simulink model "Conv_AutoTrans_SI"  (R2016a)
settings: Solver=FixedStepDiscrete  StartTime=0.0  StopTime=150  FixedStep=0.05  RelTol=1e-3
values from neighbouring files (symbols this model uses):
  VM = 1400    [initVehicle.m]
  WR = 0.25    [initVehicle.m]    (also in initWheel.m)
undefined symbols (not defined in the file or in its folder): Torque
libraries: libAutoTrans x3, libEngine x2, libWheel x1

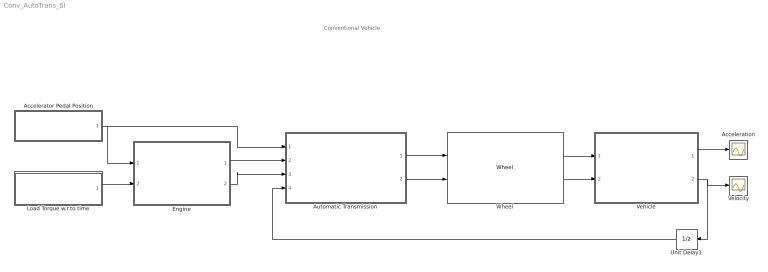
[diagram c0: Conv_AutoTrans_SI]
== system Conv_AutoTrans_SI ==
  note: Conventional Vehicle
  Acceleration : Scope
  Accelerator Pedal Position : Subsystem
  Automatic Transmission : Subsystem
  Engine : Subsystem
  Load Torque w.r.to time : Subsystem
  Unit Delay1 : UnitDelay  SampleTime=-1
  Vehicle : Subsystem
  Velocity : Scope
  Wheel : libWheel/Wheel
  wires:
  Wheel/1 -> Vehicle/1(wheel_speed)
  Wheel/2 -> Vehicle/2(propulsive_force)
  Load Torque w.r.to time/1(load_vs_time) -> Engine/2(load_vs_time)
  Vehicle/2(vehicle_velocity) -> Velocity/1, Unit Delay1/1
  Accelerator Pedal Position/1(pedal_position) -> Automatic Transmission/1(throttle_pos), Engine/1(throttle_position)
  Automatic Transmission/1(trans_speed) -> Wheel/1
  Automatic Transmission/2(trans_torque) -> Wheel/2
  Engine/1(eng_speed) -> Automatic Transmission/2(eng_speed)
  Engine/2(eng_torque) -> Automatic Transmission/3(eng_torque)
  Vehicle/1(vehicle_acceleration) -> Acceleration/1
  Unit Delay1/1 -> Automatic Transmission/4(vehicle_speed)

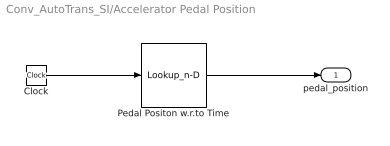
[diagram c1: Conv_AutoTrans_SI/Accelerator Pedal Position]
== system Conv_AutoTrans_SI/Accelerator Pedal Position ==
  Clock : Clock
  Pedal Positon w.r.to Time : Lookup_n-D  NumberOfTableDimensions=1  BreakpointsForDimension1=[0,20,25,35,40,60,65,75,80,100,105,115,120,140,145,155,160,180,185,195,200]  Table=[10,10,80,80,10,10,80,80,10,10,80,80,10,10,80,80,10,10,80,80,10]  RndMeth=Simplest
  pedal_position : Outport
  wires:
  Pedal Positon w.r.to Time/1 -> pedal_position/1
  Clock/1 -> Pedal Positon w.r.to Time/1

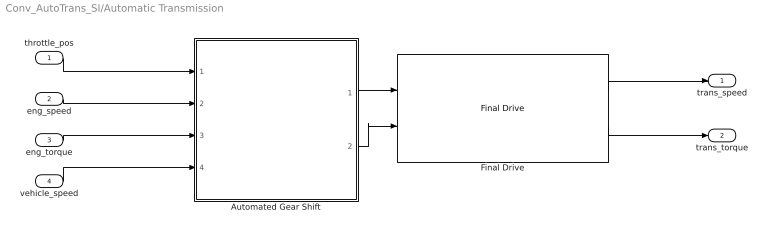
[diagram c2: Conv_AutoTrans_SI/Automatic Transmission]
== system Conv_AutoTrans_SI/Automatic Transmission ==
  throttle_pos : Inport
  eng_speed : Inport  Port=2
  eng_torque : Inport  Port=3
  vehicle_speed : Inport  Port=4
  Automated Gear Shift : Subsystem
  Final Drive : libAutoTrans/Final Drive
  trans_speed : Outport
  trans_torque : Outport  Port=2
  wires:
  Final Drive/1 -> trans_speed/1
  Final Drive/2 -> trans_torque/1
  Automated Gear Shift/1(speed_output) -> Final Drive/1
  Automated Gear Shift/2(torque_output) -> Final Drive/2
  throttle_pos/1 -> Automated Gear Shift/1(throttle_pos)
  eng_speed/1 -> Automated Gear Shift/2(eng_speed)
  eng_torque/1 -> Automated Gear Shift/3(eng_torque)
  vehicle_speed/1 -> Automated Gear Shift/4(vehicle_speed)

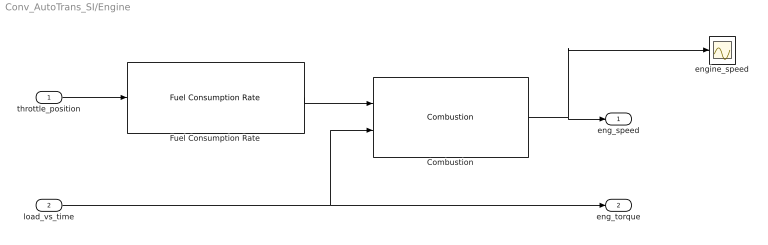
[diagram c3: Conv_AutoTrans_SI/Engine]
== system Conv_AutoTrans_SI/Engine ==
  throttle_position : Inport
  load_vs_time : Inport  Port=2
  Combustion : libEngine/Combustion
  Fuel Consumption Rate : libEngine/Fuel Consumption Rate
  engine_speed : Scope
  eng_speed : Outport
  eng_torque : Outport  Port=2
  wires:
  throttle_position/1 -> Fuel Consumption Rate/1
  Fuel Consumption Rate/1 -> Combustion/1
  load_vs_time/1 -> Combustion/2, eng_torque/1
  Combustion/1 -> engine_speed/1, eng_speed/1

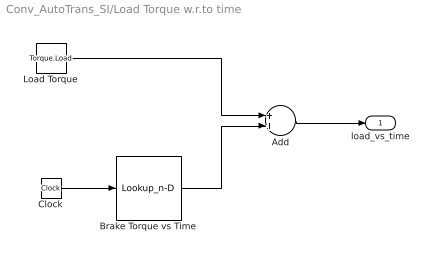
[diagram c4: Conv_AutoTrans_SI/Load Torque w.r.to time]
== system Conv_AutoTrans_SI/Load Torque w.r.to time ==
  Add : Sum
  Brake Torque vs Time : Lookup_n-D  NumberOfTableDimensions=1  BreakpointsForDimension1=[0,10,15,20,25,35,40,45,50,60,65,70,75,85,90,95,100,110,115,120,125,135,140,145,150,160,165,170,175,185,190,195,200]  Table=[0,0,2,2,0,0,2,2,0,0,2,2,0,0,2,2,0,0,2,2,0,0,2,2,0,0,2,2,0,0,2,2,0]  RndMeth=Simplest
  Clock : Clock
  Load Torque : Constant  Value=Torque.Load
  load_vs_time : Outport
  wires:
  Clock/1 -> Brake Torque vs Time/1
  Load Torque/1 -> Add/1
  Brake Torque vs Time/1 -> Add/2
  Add/1 -> load_vs_time/1

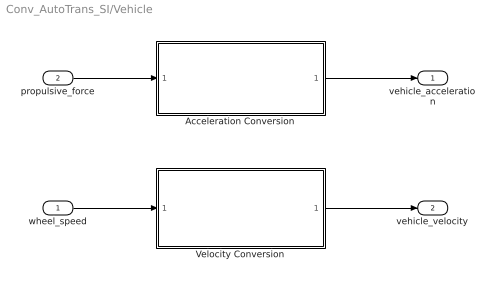
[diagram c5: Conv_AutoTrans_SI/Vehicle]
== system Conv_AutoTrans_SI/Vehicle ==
  wheel_speed : Inport
  propulsive_force : Inport  Port=2
  Acceleration Conversion : Subsystem
  Velocity Conversion : Subsystem
  vehicle_acceleration : Outport
  vehicle_velocity : Outport  Port=2
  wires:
  propulsive_force/1 -> Acceleration Conversion/1(tractive_effort)
  wheel_speed/1 -> Velocity Conversion/1(wheel_speed)
  Acceleration Conversion/1(acceleration) -> vehicle_acceleration/1
  Velocity Conversion/1(vehicle_velocity) -> vehicle_velocity/1

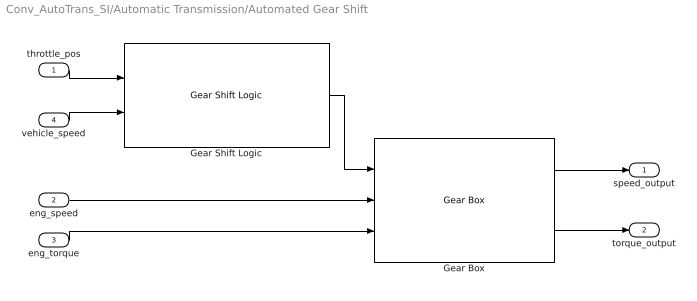
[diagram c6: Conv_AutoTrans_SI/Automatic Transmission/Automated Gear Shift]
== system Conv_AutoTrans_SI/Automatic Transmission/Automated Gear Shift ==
  throttle_pos : Inport
  eng_speed : Inport  Port=2
  eng_torque : Inport  Port=3
  vehicle_speed : Inport  Port=4
  Gear Box : libAutoTrans/Gear Box
  Gear Shift Logic : libAutoTrans/Gear Shift Logic
  speed_output : Outport
  torque_output : Outport  Port=2
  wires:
  throttle_pos/1 -> Gear Shift Logic/1
  vehicle_speed/1 -> Gear Shift Logic/2
  Gear Shift Logic/1 -> Gear Box/1
  eng_speed/1 -> Gear Box/2
  eng_torque/1 -> Gear Box/3
  Gear Box/1 -> speed_output/1
  Gear Box/2 -> torque_output/1

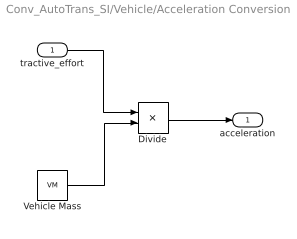
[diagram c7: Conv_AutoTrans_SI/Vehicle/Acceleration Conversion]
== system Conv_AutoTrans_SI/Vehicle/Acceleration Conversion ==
  tractive_effort : Inport
  Divide : Product  Inputs=*/
  Vehicle Mass : Constant  Value=VM
  acceleration : Outport
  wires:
  tractive_effort/1 -> Divide/1
  Vehicle Mass/1 -> Divide/2
  Divide/1 -> acceleration/1

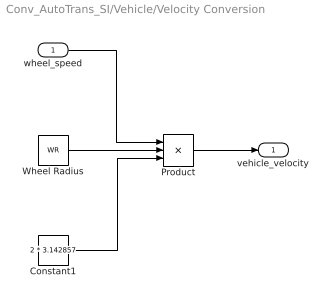
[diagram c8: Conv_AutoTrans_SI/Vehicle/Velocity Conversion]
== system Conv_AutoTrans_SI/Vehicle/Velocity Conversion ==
  wheel_speed : Inport
  Constant1 : Constant  Value=2 * 3.142857
  Product : Product  Inputs=3
  Wheel Radius : Constant  Value=WR
  vehicle_velocity : Outport
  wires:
  wheel_speed/1 -> Product/1
  Wheel Radius/1 -> Product/2
  Constant1/1 -> Product/3
  Product/1 -> vehicle_velocity/1
